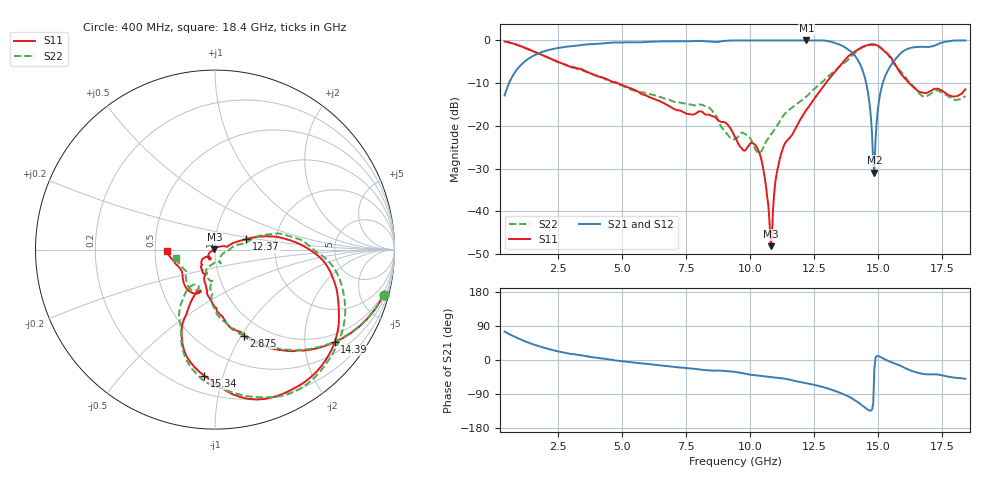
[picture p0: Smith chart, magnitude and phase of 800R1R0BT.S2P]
!  American Technical Ceramics  Date:  6/19/09
!  One Norden Lane
!  Huntington Station,  NY.  11746-2102
!  Tel:  (631) 622-4700  Fax:  (631) 622-4748
!  Part Number  800R1R0BT
!  Description: Ultra-low ESR, NPO  Mounting Orientation: Horizontal
!  Application: High RF power Filters, Combiners, Matching networks,
!  Antenna, DC block, Bypass and Couplers
# GHZ S DB R 50
! Freq  |S11|  S11 Ph  |S21|  S21 Ph  |S12|  S12 Ph  |S22|  S22 Ph
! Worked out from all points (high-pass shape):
!   401 points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, 400 MHz to 18.4 GHz, reference 50 ohm
!   highest |S21| = -0.01 dB at 12.19 GHz (marker M1); lowest = -30.9 dB at 14.85 GHz (marker M2)
!   |S21| within 3 dB of the highest: 1.735 GHz to 14 GHz (12.27 GHz wide, 156 % of centre); 15.87 GHz to end of sweep
!   lowest |S11| = -48.1 dB at 10.79 GHz (marker M3), VSWR 1.01, Z = 49.7 + j0.196 ohm
!   |S11| at or under -10 dB: 4.807 GHz to 12.95 GHz (8.143 GHz wide, 91.7 % of centre); 16.21 GHz to end of sweep
!   |S22| runs from -26.4 to -0.2 dB; largest |S21 - S12| = 0.0027
!   S11 on the Smith chart (normalised r, x): 400 MHz: 0.79, -7.47; 2.875 GHz: 0.80, -1.02; 12.37 GHz: 1.41, +0.17; 14.39 GHz: 0.77, -2.74; 15.34 GHz: 0.31, -0.87; 18.4 GHz: 0.58, -0.01
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0.4  -0.24 -15.1  -12.88 74.8  -12.89 74.8  -0.23 -15.0
1.345  -2.09 -44.6  -4.22 45.4  -4.22 45.4  -2.11 -44.2
2.875  -5.93 -71.6  -1.43 17.4  -1.43 17.4  -5.98 -71.0
3.415  -6.76 -77.0  -1.07 12.3  -1.07 12.3  -6.94 -77.5
6.43  -14.13 -106.3  -0.23 -13.9  -0.23 -13.9  -13.12 -96.8
8.365  -17.36 -121.6  -0.24 -27.4  -0.24 -27.5  -15.65 -104.0
9.4  -22.62 -142.5  -0.01 -31.4  -0.01 -31.4  -23.06 -75.4
10.3  -25.65 -136.2  -0.01 -41.1  -0.01 -41.1  -26.41 -43.9
10.525  -30.80 -152.1  -0.01 -42.8  -0.01 -42.8  -24.83 -14.1
10.795  -48.15 149.8  -0.01 -45.0  -0.01 -45.0  -22.04 -1.1
11.245  -25.73 21.8  -0.01 -48.3  -0.01 -48.3  -18.01 12.3
12.19  -16.26 19.0  -0.01 -61.5  -0.01 -61.6  -13.14 16.5
12.37  -14.73 18.5  -0.01 -63.8  -0.01 -63.8  -12.05 17.5
12.415  -14.39 18.3  -0.01 -64.4  -0.01 -64.4  -11.79 17.2
13.54  -5.65 0.3  -1.12 -87.5  -1.12 -87.6  -5.82 3.7
14.395  -1.48 -37.7  -7.18 -121.4  -7.18 -121.4  -1.59 -30.7
14.845  -1.03 -64.8  -30.91 -21.9  -30.92 -21.6  -0.88 -62.9
15.07  -1.60 -80.5  -12.57 8.4  -12.57 8.4  -1.68 -79.5
15.34  -3.03 -94.9  -7.41 -1.3  -7.41 -1.3  -3.02 -98.0
15.43  -3.57 -100.0  -6.41 -3.8  -6.43 -3.8  -3.77 -103.5
16.6  -12.05 -111.9  -1.52 -34.8  -1.53 -34.8  -12.42 -122.9
18.4  -11.46 -177.9  -0.01 -49.7  -0.01 -49.7  -13.05 -167.8
